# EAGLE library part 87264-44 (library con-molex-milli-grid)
RECEPTACAL
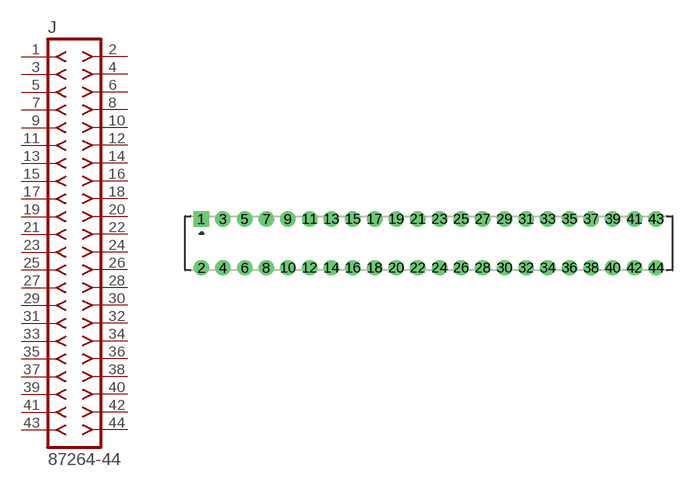
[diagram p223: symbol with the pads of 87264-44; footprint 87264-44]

Designator prefix J

## 87264-44  [87264-44]
1  1  pas
2  2  pas
3  3  pas
4  4  pas
5  5  pas
6  6  pas
7  7  pas
8  8  pas
9  9  pas
10  10  pas
11  11  pas
12  12  pas
13  13  pas
14  14  pas
15  15  pas
16  16  pas
17  17  pas
18  18  pas
19  19  pas
20  20  pas
21  21  pas
22  22  pas
23  23  pas
24  24  pas
25  25  pas
26  26  pas
27  27  pas
28  28  pas
29  29  pas
30  30  pas
31  31  pas
32  32  pas
33  33  pas
34  34  pas
35  35  pas
36  36  pas
37  37  pas
38  38  pas
39  39  pas
40  40  pas
41  41  pas
42  42  pas
43  43  pas
44  44  pas

## Footprint 87264-44 (pad centres in mm)
RECEPTACAL Dual Row, Side Entry
drill 0.914 square: 1 -21,2.25
drill 0.914: 2 -21,-2.25; 3 -19,2.25; 4 -19,-2.25; 5 -17,2.25; 6 -17,-2.25; 7 -15,2.25; 8 -15,-2.25; 9 -13,2.25; 10 -13,-2.25; 11 -11,2.25; 12 -11,-2.25; 13 -9,2.25; 14 -9,-2.25; 15 -7,2.25; 16 -7,-2.25; 17 -5,2.25; 18 -5,-2.25; 19 -3,2.25; 20 -3,-2.25; 21 -1,2.25; 22 -1,-2.25; 23 1,2.25; 24 1,-2.25; 25 3,2.25; 26 3,-2.25; 27 5,2.25; 28 5,-2.25; 29 7,2.25; 30 7,-2.25; 31 9,2.25; 32 9,-2.25; 33 11,2.25; 34 11,-2.25; 35 13,2.25; 36 13,-2.25; 37 15,2.25; 38 15,-2.25; 39 17,2.25; 40 17,-2.25; 41 19,2.25; 42 19,-2.25; 43 21,2.25; 44 21,-2.25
